PROGRAM MAIN
VAR
	master,slave:				axis_ref;
	power_m,power_s:		MC_Power;
	process:					step;
	move_m:				MC_MoveVelocity;
	move_s:					MC_MoveModulo;
	stop_m:					MC_Stop;
	setpos_m:				MC_SetPosition;
	reset_s,reset_m:			MC_Reset;

	bEL1259_input AT%I*:	BOOL;

	camin:					MC_CamIn;
	camout:					MC_CamOut;
	camtableselect:			MC_CamTableSelect;
	cam_table1:				MC_CAM_REF;
	table1:					ARRAY[1..4]OF MC_MotionFunctionPoint;

END_VAR

axis_basic();
cam();
master();
slave();
CASE process OF
init:
	reset_m.Execute:=FALSE;
	reset_s.Execute:=FALSE;
	camin.Execute:=FALSE;
	move_m.Execute:=FALSE;
	move_s.Execute:=FALSE;
	camout.Execute:=FALSE;
	IF power_m.status AND power_s.status THEN
		process:=homing;
	END_IF
	IF slave.Status.Error OR master.Status.Error THEN
		process:=error;
	END_IF

homing:
	move_m.Execute:=TRUE;
	move_s.Execute:=TRUE;
	IF move_m.InVelocity AND	bEL1259_input  THEN
		stop_m.Execute:=TRUE;
	END_IF
	IF stop_m.Done AND move_s.Done THEN
		setpos_m.Execute:=TRUE;
		move_m.Execute:=FALSE;
		move_s.Execute:=FALSE;
		stop_m.Execute:=FALSE;
		IF	setpos_m.Done THEN
			setpos_m.Execute:=FALSE;
			process:=creating_cam;
		END_IF
	END_IF
	IF slave.Status.Error OR master.Status.Error THEN
		process:=error;
	END_IF

creating_cam:
	camtableselect.Execute:=TRUE;
	IF camtableselect.Done THEN
		camtableselect.Execute:=FALSE;
		move_m.Execute:=TRUE;
		IF master.Status.Moving THEN
			process:=camming;
			move_m.Execute:=FALSE;
		END_IF
	END_IF
	IF slave.Status.Error OR master.Status.Error THEN
		process:=error;
	END_IF

camming:
	camout.Execute:=false;
	camin.Execute:=bEL1259_input ;

	IF camin.InSync THEN
		process:=InSync;
	END_IF
	IF slave.Status.Error OR master.Status.Error THEN
		process:=error;
	END_IF

InSync:
	(*IF   slave.NcToPlc.ActPos <0.1 OR slave.NcToPlc.ActPos>16.63 THEN*)
	IF NOT slave.Status.Moving THEN
		camout.Execute:=TRUE;
		IF camout.Done THEN
			process:=camming;
		END_IF
	END_IF
	IF slave.Status.Error OR master.Status.Error THEN
		process:=error;
	END_IF

error:
	camout.Execute:=slave.Status.Coupled;
	IF NOT slave.Status.Coupled THEN
		IF master.Status.Error OR slave.Status.Error THEN
			process:=reset;
		ELSE
			process:=init;
		END_IF
	END_IF

reset:
	reset_m.Execute:=TRUE;
	reset_s.Execute:=TRUE;
	camin.Execute:=FALSE;
	move_m.Execute:=FALSE;
	move_s.Execute:=FALSE;
	IF reset_m.Done AND reset_s.Done THEN
		process:=init;
	ELSIF reset_m.Error OR reset_s.Error THEN
		process:=init;
	END_IF





END_CASE

ACTION axis_basic:
power_m(
	Enable:=TRUE ,
	Enable_Positive:= TRUE,
	Enable_Negative:=TRUE ,
	Axis:=master , );
power_S(
	Enable:=TRUE ,
	Enable_Positive:= TRUE,
	Enable_Negative:=TRUE ,
	Axis:=slave , );
move_m(
	Execute:=move_m.Execute ,
	Velocity:=300 ,
	Direction:=1 ,
	Axis:=master , );
move_s(
	Execute:=move_s.Execute ,
	Position:=239 ,
	Velocity:=300,
	Axis:=slave , );
setpos_m(
	Execute:= setpos_m.Execute,
	Position:= 0,
	Axis:= master, );
stop_m(
	Execute:=stop_m.Execute ,
	Axis:=master ,);
reset_m(
	Execute:=reset_m.Execute ,
	Axis:=master , );
reset_s(
	Execute:=reset_s.Execute ,
	Axis:=slave , );
END_ACTION

ACTION cam:
camin(
	Execute:=camin.Execute ,
	StartMode:= MC_STARTMODE_relative,
	CamTableID:=1 ,
	Master:= master,
	Slave:=slave , );
camout(
	Execute:=camout.Execute ,
	Slave:=slave , );
camtableselect(
	Execute:=camtableselect.Execute ,
	Periodic:=FALSE ,
	MasterAbsolute:= ,
	SlaveAbsolute:= ,
	CamTableID:= 1,
	Master:=master ,
	Slave:=slave ,
	CamTable:= cam_table1, );

cam_table1.ArraySize:=SIZEOF(table1);
cam_table1.NoOfColumns:=1;
cam_table1.NoOfRows:=4;
cam_table1.pArray:=ADR(table1);
cam_table1.TableType:=22;(*MC_TableType_TABULARTYPE_MOTIONFUNC*)

table1[1].FunctionType:=MOTIONFUNCTYPE_POLYNOM1;
table1[1].MasterPos:=0;
table1[1].SlavePos:=0;
table1[1].PointIndex:=1;
table1[1].PointType:=MOTIONPOINTTYPE_REST;

table1[2].FunctionType:=MOTIONFUNCTYPE_POLYNOM1;
table1[2].MasterPos:=170.3;
table1[2].SlavePos:=55.75;
table1[2].PointIndex:=2;
table1[2].PointType:=MOTIONPOINTTYPE_VELOCITY;
table1[2].SlaveVelo:=300;

table1[3].FunctionType:=MOTIONFUNCTYPE_POLYNOM5;
table1[3].MasterPos:=179.3;
table1[3].SlavePos:=60.75;
table1[3].PointIndex:=3;
table1[3].PointType:=MOTIONPOINTTYPE_VELOCITY;
table1[3].SlaveVelo:=300;

table1[4].FunctionType:=MOTIONFUNCTYPE_POLYNOM3;
table1[4].MasterPos:=357.55;
table1[4].SlavePos:=239;
table1[4].PointIndex:=4;
table1[4].PointType:=MOTIONPOINTTYPE_REST;
END_ACTION

END_PROGRAM
